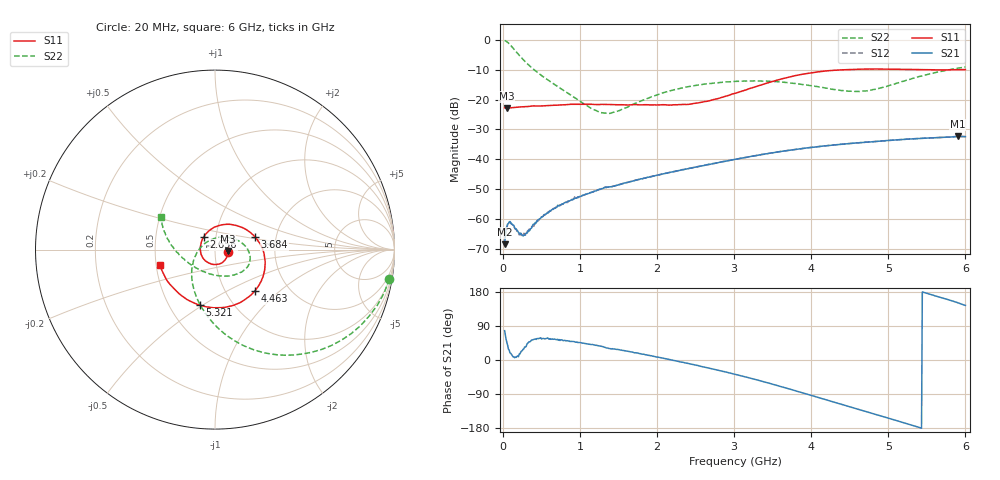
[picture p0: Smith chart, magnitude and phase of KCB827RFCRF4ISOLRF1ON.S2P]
!Agilent Technologies,E5071B,JP1KK00126,A.08.11
!Date: Tue May 06 07:14:54 2014
!Data & Calibration Information:
!Freq	S11:SOLT2(ON)	S21:SOLT2(ON)	S12:SOLT2(ON)	S22:SOLT2(ON)
# Hz S dB R 50
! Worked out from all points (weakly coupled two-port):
!   600 points, 20 MHz to 6 GHz, reference 50 ohm
!   highest |S21| = -32.33 dB at 5.9 GHz (marker M1); lowest = -68.6 dB at 20 MHz (marker M2)
!   lowest |S11| = -22.8 dB at 49.95 MHz (marker M3), VSWR 1.16, Z = 57.7 - j0.904 ohm
!   |S11| at or under -10 dB: start of sweep to 4.385 GHz; 5.653 GHz to 5.758 GHz (105 MHz wide, 1.84 % of centre)
!   |S22| runs from -24.6 to -0.1 dB; largest |S21 - S12| = 0.00015
!   S11 on the Smith chart (normalised r, x): 20 MHz: 1.15, -0.03; 2.656 GHz: 0.87, +0.12; 3.684 GHz: 1.55, +0.23; 4.463 GHz: 1.36, -0.70; 5.321 GHz: 0.71, -0.49; 6 GHz: 0.52, -0.10
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2e7  -22.76 -11.5  -68.62 77.3  -69.19 78.5  -0.12 -9.6
4.994992e7  -22.84 -6.2  -62.70 46.4  -62.69 43.2  -0.58 -23.3
8.988314e7  -22.76 -6.7  -60.92 18.8  -61.11 19.5  -1.51 -39.5
1.397997e8  -22.64 -8.9  -62.22 8.2  -62.21 7.8  -2.99 -56.1
2.296494e8  -22.41 -13.9  -64.79 20.9  -65.32 17.5  -5.67 -77.7
3.194992e8  -22.31 -21.1  -64.51 44.4  -64.00 44.5  -8.05 -93.2
4.692487e8  -22.16 -30.7  -60.15 57.1  -60.37 57.6  -11.32 -113.6
6.289816e8  -21.92 -43.2  -56.99 54.9  -56.89 55.7  -14.22 -131.9
1.018331e9  -21.55 -72.6  -52.36 45.3  -52.25 45.2  -20.90 -179.0
1.247947e9  -21.65 -91.3  -50.09 37.3  -50.16 36.3  -24.18 138.3
1.37773e9  -21.62 -101.8  -49.31 30.3  -49.26 30.3  -24.63 109.7
2.016661e9  -21.78 -157.6  -45.28 7.3  -45.28 7.0  -18.25 28.7
2.655593e9  -20.52 131.6  -41.81 -20.7  -41.85 -20.9  -14.64 -1.1
3.014992e9  -17.85 88.1  -40.04 -37.9  -40.01 -38.1  -13.87 -14.6
3.683873e9  -12.62 17.3  -37.09 -74.7  -37.10 -74.9  -14.23 -40.2
4.013322e9  -10.93 -11.4  -36.00 -94.4  -35.98 -94.3  -15.41 -58.1
4.462571e9  -9.89 -46.3  -34.82 -121.3  -34.80 -121.4  -17.11 -96.6
4.722137e9  -9.71 -64.5  -34.26 -136.8  -34.27 -136.9  -16.99 -127.2
5.011653e9  -9.75 -83.5  -33.70 -154.0  -33.68 -154.2  -15.22 -158.1
5.321135e9  -9.88 -105.0  -33.15 -173.0  -33.12 -173.2  -12.82 178.7
5.900167e9  -9.96 -154.4  -32.33 150.9  -32.31 150.8  -9.40 152.2
6e9  -9.90 -164.2  -32.43 144.1  -32.41 144.2  -9.05 149.0
